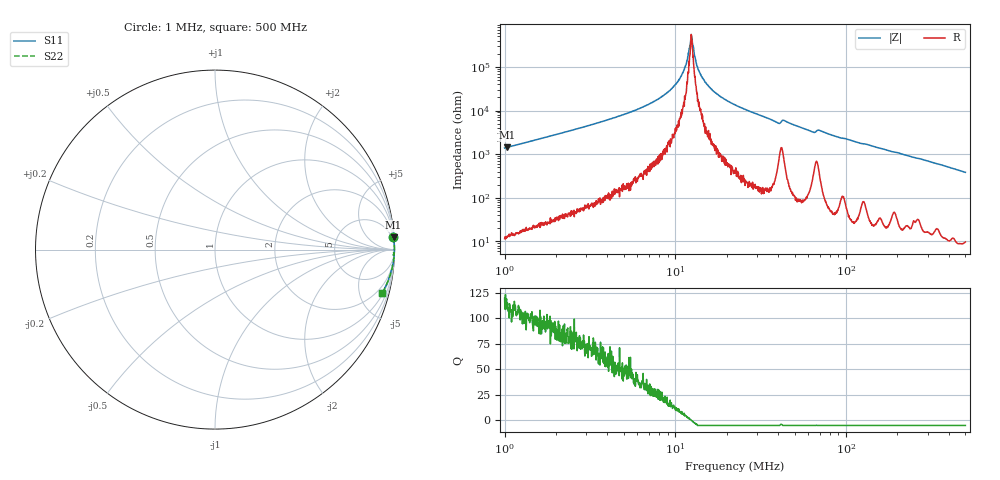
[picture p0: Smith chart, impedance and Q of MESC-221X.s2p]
!s-Parameter Generated by FASTRON Sdn. Bhd.
!FASTRON P/N : MESC-221X
!Keysight Technologies,E4991B,MY54100416,A.01.15
!Date: Fri Mar 27 11:22:51 2026
!Version  : Rev00 Fri Mar 27 11:22:51 2026
!Data & Calibration Information:
!PortZ  Port1:50+j0  Port2:50+j0
!When reading, reference impedance value at option line is always used.
!Remarks : This data is being provided solely for informational purposes.
!Freq	S11	S21	S12	S22
# Hz S dB R 50
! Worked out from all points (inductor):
!   1601 points, 1 MHz to 500 MHz, reference 50 ohm
!   read as one part in series: L = 218 uH near 1.032 MHz
!   highest Q = 112 at 1.04 MHz (marker M1), where L = 220 uH
!   self-resonance near 12.34 MHz
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1000000  -0.03 4.1  -22.84 -85.4  -22.84 -85.4  -0.03 4.1
1039605  -0.03 4.0  -23.18 -85.5  -23.18 -85.5  -0.03 4.0
2820919  -0.01 1.4  -32.18 -87.8  -32.18 -87.8  -0.01 1.4
5354537  -0.00 0.6  -39.01 -88.4  -39.01 -88.4  -0.00 0.6
7957584  -0.00 0.3  -45.34 -87.1  -45.34 -87.1  -0.00 0.3
9367619  -0.00 0.2  -49.52 -85.5  -49.52 -85.5  -0.00 0.2
1.060739e7  -0.00 0.1  -54.50 -83.0  -54.50 -83.0  -0.00 0.1
1.141981e7  -0.00 0.1  -60.31 -78.8  -60.31 -78.8  -0.00 0.1
1.215202e7  -0.00 0.0  -69.52 -53.1  -69.52 -53.1  -0.00 0.0
1.243855e7  -0.00 -0.0  -74.29 9.0  -74.29 9.0  -0.00 -0.0
1.268247e7  -0.00 -0.0  -69.36 55.3  -69.36 55.3  -0.00 -0.0
1.323608e7  -0.00 -0.0  -61.74 73.0  -61.74 73.0  -0.00 -0.0
1.365382e7  -0.00 -0.1  -58.67 79.9  -58.67 79.9  -0.00 -0.1
1.492973e7  -0.00 -0.1  -53.00 84.6  -53.00 84.6  -0.00 -0.1
1.750705e7  -0.00 -0.2  -47.54 86.5  -47.54 86.5  -0.00 -0.2
2.236068e7  -0.00 -0.4  -42.59 87.9  -42.59 87.9  -0.00 -0.4
3.973194e7  -0.02 -1.1  -34.36 83.6  -34.36 83.6  -0.02 -1.1
4.361384e7  -0.02 -1.0  -35.37 83.2  -35.37 83.2  -0.02 -1.0
6.307767e7  -0.02 -1.7  -30.31 84.3  -30.31 84.3  -0.02 -1.7
7.005203e7  -0.03 -1.6  -30.89 83.2  -30.89 83.2  -0.03 -1.6
1.77937e8  -0.04 -4.8  -21.62 84.1  -21.62 84.1  -0.04 -4.8
5e8  -0.34 -14.5  -12.01 74.0  -12.01 74.0  -0.34 -14.5
